| IBIS file stm32u535_545_ufbga64.ibs
[IBIS ver] 4.2
[File name] stm32u535_545_ufbga64.ibs
[File Rev] rev1.0
[Date]  11-09-2023
[Source] Data Created at STMicroelectronics
[Notes]  File originated from ELDO simulations.
[Disclaimer]  This information is for modeling purpose only and is
   not guaranteed. The information is subject to change without
   notice.
[Copyright] Copyright 2023 STMicroelectronics Inc.
|   Component stm32u535_545_ufbga64
[Component] stm32u535_545_ufbga64
[Manufacturer] STMicroelectronics
[Package]
| variable   typ   min   max
R_pkg  0  NA  NA
L_pkg  0  NA  NA
C_pkg  0  NA  NA
[Pin]   signal_name   model_name
A1  PC14-OSC32_IN   io8_100m_tamp_ft
A2  PC13  io8_100m_ft_v33
A3  PB9  io8_100m_hslv_i2c_ft
A4  PB4  io8_100m_i2c_ft
A5  PB3  io8_100m_i2c_ft
A6  PA15  io8_100m_ft
A7  PA14  io8_100m_ft
A8  PA13  io8_100m_ft
B1  PC15-OSC32_OUT  io8_100m_tamp_ft
B2  VBAT  power
B3  PB8  io8_100m_hslv_i2c_ft
B4  PH3-BOOT0  io8_100m_ft
B5  PD2  io8_100m_hslv_ft
B6  PC11  io8_100m_hslv_ft
B7  PC10  io8_100m_hslv_ft
B8  PA12  io8_usb_ft
C1  PH0-OSC_IN  io8_100m_ft
C2  VSS  gnd
C3  PB7  io8_166m_hslv_i2c_ft
C4  PB5  io8_166m_hslv_ft
C5  PC12  io8_166m_hslv_ft
C6  PA10  io8_100m_ft
C7  PA9  io8_100m_ft
C8  PA11  io8_usb_ft
D1  PH1-OSC_OUT  io8_100m_ft
D2  VDD  power
D3  PB6  io8_100m_i2c_ft
D4  VSS  gnd
D5  VSS  gnd
D6  VSS  gnd
D7  PA8  io8_166m_hslv_ft
D8  PC9  io8_100m_hslv_ft
E1  NRST  nc
E2  PC1  io8_166m_hslv_i2c_ft
E3  PC0  io8_100m_hslv_i2c_ft
E4  VDD  power
E5  VDDUSB  power
E6  VDD  power
E7  PC7  io8_100m_hslv_ft
E8  PC8  io8_100m_hslv_ft
F1  VSSA  nc
F2  PC2  io8_100m_hslv_ft
F3  PA2  io8_100m_hslv_ft
F4  PA5  io8_100m_ft
F5  PB0  io8_100m_hslv_ft
F6  PC6  io8_100m_hslv_ft
F7  PB15  io8_100m_ft
F8  PB14  io8_100m_i2c_ft
G1  PC3  io8_100m_hslv_ft
G2  PA0  io8_100m_hslv_tamp_ft
G3  PA3  io8_166m_hslv_ft
G4  PA6  io8_100m_hslv_ft
G5  PB1  io8_100m_hslv_ft
G6  PB2  io8_100m_hslv_tamp_ft
G7  PB10  io8_166m_hslv_i2c_ft
G8  PB13  io8_100m_i2c_ft
H1  VDDA  power
H2  PA1  io8_100m_hslv_tamp_ft
H3  PA4  io8_100m_hslv_ft
H4  PA7  io8_100m_hslv_i2c_ft
H5  PC4  io8_100m_hslv_ft
H6  PC5  io8_100m_tamp_ft
H7  VCAP  nc
H8  PB12  io8_166m_hslv_ft
[Package Model]   455-ufbga-5x5-64ldo-100mhz-230421
[Pin Mapping]   pulldown_ref   pullup_ref   | Comment
A1  gndio  vddiom  | Depending on IO usage
| A1  gndio  vsw  | Depending on IO usage
A2  gndio  vddiom  | Depending on IO usage
| A2  gndio  vsw  | Depending on IO usage
A3  gndio  vddiom
A4  gndio  vddiom
A5  gndio  vddiom
A6  gndio  vddiom
A7  gndio  vddiom
A8  gndio  vddiom  | Depending on IO usage
| A8  gndio  vddusb  | Depending on IO usage
B1  gndio  vddiom  | Depending on IO usage
| B1  gndio  vsw  | Depending on IO usage
B2  nc  vsw
B3  gndio  vddiom
B4  gndio  vddiom
B5  gndio  vddiom
B6  gndio  vddiom
B7  gndio  vddiom
B8  gndio  vddiom  | Depending on IO usage
| B8  gndio  vddusb  | Depending on IO usage
C1  gndio  vddiom
C2  gndio  nc
C3  gndio  vddiom
C4  gndio  vddiom
C5  gndio  vddiom
C6  gndio  vddiom  | Depending on IO usage
| C6  gndio  vddusb  | Depending on IO usage
C7  gndio  vddiom  | Depending on IO usage
| C7  gndio  vddusb  | Depending on IO usage
C8  gndio  vddiom  | Depending on IO usage
| C8  gndio  vddusb  | Depending on IO usage
D1  gndio  vddiom
D2  nc  vddiom
D3  gndio  vddiom
D4  gndio  nc
D5  gndio  nc
D6  gndio  nc
D7  gndio  vddiom
D8  gndio  vddiom
E1  nc   nc
E2  gndio  vddiom
E3  gndio  vddiom
E4  nc  vddiom
E5  nc  vddusb
E6  nc  vddiom
E7  gndio  vddiom
E8  gndio  vddiom
F1  nc  nc
F2  gndio  vddiom
F3  gndio  vddiom
F4  gndio  vddiom
F5  gndio  vddiom
F6  gndio  vddiom
F7  gndio  vddiom
F8  gndio  vddiom
G1  gndio  vddiom
G2  gndio  vddiom
G3  gndio  vddiom
G4  gndio  vddiom
G5  gndio  vddiom
G6  gndio  vddiom
G7  gndio  vddiom
G8  gndio  vddiom
H1  nc  vddiom
H2  gndio  vddiom
H3  gndio  vddiom
H4  gndio  vddiom
H5  gndio  vddiom
H6  gndio  vddiom
H7  nc  nc
H8  gndio  vddiom
[Model Selector] io8_100m_ft
io8_100m_ft_hs_1v2  "IO8_FT 100MHz high speed @ 1.2V"
io8_100m_ft_fs_1v2  "IO8_FT 100MHz fast speed @ 1.2V"
io8_100m_ft_fs_pd_1v2  "IO8_FT 100MHz fast speed @ 1.2V pulldown"
io8_100m_ft_ms_1v2  "IO8_FT 100MHz med speed @ 1.2V"
io8_100m_ft_ms_pd_1v2  "IO8_FT 100MHz med speed @ 1.2V pulldown"
io8_100m_ft_ls_1v2  "IO8_FT 100MHz low speed @ 1.2V"
io8_100m_ft_ls_pd_1v2  "IO8_FT 100MHz low speed @ 1.2V pulldown"
io8_100m_ft_hs_1v8  "IO8_FT 100MHz high speed @ 1.8V"
io8_100m_ft_hs_pd_1v8  "IO8_FT 100MHz high speed @ 1.8V pulldown"
io8_100m_ft_fs_1v8  "IO8_FT 100MHz fast speed @ 1.8V"
io8_100m_ft_fs_pd_1v8  "IO8_FT 100MHz fast speed @ 1.8V pulldown"
io8_100m_ft_ms_1v8  "IO8_FT 100MHz med speed @ 1.8V"
io8_100m_ft_ms_pd_1v8  "IO8_FT 100MHz med speed @ 1.8V pulldown"
io8_100m_ft_ls_1v8  "IO8_FT 100MHz low speed @ 1.8V"
io8_100m_ft_ls_pd_1v8  "IO8_FT 100MHz low speed @ 1.8V pulldown"
io8_100m_ft_hs_3v3  "IO8_FT 100MHz high speed @ 3.3V"
io8_100m_ft_hs_pd_3v3  "IO8_FT 100MHz high speed @ 3.3V pulldown"
io8_100m_ft_fs_3v3  "IO8_FT 100MHz fast speed @ 3.3V"
io8_100m_ft_fs_pd_3v3  "IO8_FT 100MHz fast speed @ 3.3V pulldown"
io8_100m_ft_ms_3v3  "IO8_FT 100MHz med speed @ 3.3V"
io8_100m_ft_ms_pd_3v3  "IO8_FT 100MHz med speed @ 3.3V pulldown"
io8_100m_ft_ls_3v3  "IO8_FT 100MHz low speed @ 3.3V"
io8_100m_ft_ls_pd_3v3  "IO8_FT 100MHz low speed @ 3.3V pulldown"
[Model Selector] io8_100m_hslv_ft
io8_100m_ft_hs_1v2  "IO8_FT 100MHz high speed @ 1.2V"
io8_100m_ft_hs_pu_1v2  "IO8_FT 100MHz high speed @ 1.2V pullup"
io8_100m_ft_hs_pd_1v2  "IO8_FT 100MHz high speed @ 1.2V pulldown"
io8_100m_ft_fs_1v2  "IO8_FT 100MHz fast speed @ 1.2V"
io8_100m_ft_fs_pu_1v2  "IO8_FT 100MHz fast speed @ 1.2V pullup"
io8_100m_ft_fs_pd_1v2  "IO8_FT 100MHz fast speed @ 1.2V pulldown"
io8_100m_ft_ms_1v2  "IO8_FT 100MHz med speed @ 1.2V"
io8_100m_ft_ms_pu_1v2  "IO8_FT 100MHz med speed @ 1.2V pullup"
io8_100m_ft_ms_pd_1v2  "IO8_FT 100MHz med speed @ 1.2V pulldown"
io8_100m_ft_ls_1v2  "IO8_FT 100MHz low speed @ 1.2V"
io8_100m_ft_ls_pu_1v2  "IO8_FT 100MHz low speed @ 1.2V pullup"
io8_100m_ft_ls_pd_1v2  "IO8_FT 100MHz low speed @ 1.2V pulldown"
io8_100m_ft_hs_1v8  "IO8_FT 100MHz high speed @ 1.8V"
io8_100m_ft_hs_pu_1v8  "IO8_FT 100MHz high speed @ 1.8V pullup"
io8_100m_ft_hs_pd_1v8  "IO8_FT 100MHz high speed @ 1.8V pulldown"
io8_100m_ft_fs_1v8  "IO8_FT 100MHz fast speed @ 1.8V"
io8_100m_ft_fs_pu_1v8  "IO8_FT 100MHz fast speed @ 1.8V pullup"
io8_100m_ft_fs_pd_1v8  "IO8_FT 100MHz fast speed @ 1.8V pulldown"
io8_100m_ft_ms_1v8  "IO8_FT 100MHz med speed @ 1.8V"
io8_100m_ft_ms_pu_1v8  "IO8_FT 100MHz med speed @ 1.8V pullup"
io8_100m_ft_ms_pd_1v8  "IO8_FT 100MHz med speed @ 1.8V pulldown"
io8_100m_ft_ls_1v8  "IO8_FT 100MHz low speed @ 1.8V"
io8_100m_ft_ls_pu_1v8  "IO8_FT 100MHz low speed @ 1.8V pullup"
io8_100m_ft_ls_pd_1v8  "IO8_FT 100MHz low speed @ 1.8V pulldown"
io8_100m_ft_hs_3v3  "IO8_FT 100MHz high speed @ 3.3V"
io8_100m_ft_hs_pu_3v3  "IO8_FT 100MHz high speed @ 3.3V pullup"
io8_100m_ft_hs_pd_3v3  "IO8_FT 100MHz high speed @ 3.3V pulldown"
io8_100m_ft_fs_3v3  "IO8_FT 100MHz fast speed @ 3.3V"
io8_100m_ft_fs_pu_3v3  "IO8_FT 100MHz fast speed @ 3.3V pullup"
io8_100m_ft_fs_pd_3v3  "IO8_FT 100MHz fast speed @ 3.3V pulldown"
io8_100m_ft_ms_3v3  "IO8_FT 100MHz med speed @ 3.3V"
io8_100m_ft_ms_pu_3v3  "IO8_FT 100MHz med speed @ 3.3V pullup"
io8_100m_ft_ms_pd_3v3  "IO8_FT 100MHz med speed @ 3.3V pulldown"
io8_100m_ft_ls_3v3  "IO8_FT 100MHz low speed @ 3.3V"
io8_100m_ft_ls_pu_3v3  "IO8_FT 100MHz low speed @ 3.3V pullup"
io8_100m_ft_ls_pd_3v3  "IO8_FT 100MHz low speed @ 3.3V pulldown"
io8_100m_hslv_ft_hs_1v2  "IO8_FT 100MHz HSLV high speed @ 1.2V"
io8_100m_hslv_ft_hs_pu_1v2  "IO8_FT 100MHz HSLV high speed @ 1.2V pullup"
io8_100m_hslv_ft_hs_pd_1v2  "IO8_FT 100MHz HSLV high speed @ 1.2V pulldown"
io8_100m_hslv_ft_fs_1v2  "IO8_FT 100MHz HSLV fast speed @ 1.2V"
io8_100m_hslv_ft_fs_pu_1v2  "IO8_FT 100MHz HSLV fast speed @ 1.2V pullup"
io8_100m_hslv_ft_fs_pd_1v2  "IO8_FT 100MHz HSLV fast speed @ 1.2V pulldown"
io8_100m_hslv_ft_ms_1v2  "IO8_FT 100MHz HSLV med speed @ 1.2V"
io8_100m_hslv_ft_ms_pu_1v2  "IO8_FT 100MHz HSLV med speed @ 1.2V pullup"
io8_100m_hslv_ft_ms_pd_1v2  "IO8_FT 100MHz HSLV med speed @ 1.2V pulldown"
io8_100m_hslv_ft_ls_1v2  "IO8_FT 100MHz HSLV low speed @ 1.2V"
io8_100m_hslv_ft_ls_pu_1v2  "IO8_FT 100MHz HSLV low speed @ 1.2V pullup"
io8_100m_hslv_ft_ls_pd_1v2  "IO8_FT 100MHz HSLV low speed @ 1.2V pulldown"
io8_100m_hslv_ft_hs_1v8  "IO8_FT 100MHz HSLV high speed @ 1.8V"
io8_100m_hslv_ft_hs_pu_1v8  "IO8_FT 100MHz HSLV high speed @ 1.8V pullup"
io8_100m_hslv_ft_hs_pd_1v8  "IO8_FT 100MHz HSLV high speed @ 1.8V pulldown"
io8_100m_hslv_ft_fs_1v8  "IO8_FT 100MHz HSLV fast speed @ 1.8V"
io8_100m_hslv_ft_fs_pu_1v8  "IO8_FT 100MHz HSLV fast speed @ 1.8V pullup"
io8_100m_hslv_ft_fs_pd_1v8  "IO8_FT 100MHz HSLV fast speed @ 1.8V pulldown"
io8_100m_hslv_ft_ms_1v8  "IO8_FT 100MHz HSLV med speed @ 1.8V"
io8_100m_hslv_ft_ms_pu_1v8  "IO8_FT 100MHz HSLV med speed @ 1.8V pullup"
io8_100m_hslv_ft_ms_pd_1v8  "IO8_FT 100MHz HSLV med speed @ 1.8V pulldown"
io8_100m_hslv_ft_ls_1v8  "IO8_FT 100MHz HSLV low speed @ 1.8V"
io8_100m_hslv_ft_ls_pu_1v8  "IO8_FT 100MHz HSLV low speed @ 1.8V pullup"
io8_100m_hslv_ft_ls_pd_1v8  "IO8_FT 100MHz HSLV low speed @ 1.8V pulldown"
io8_100m_hslv_ft_hs_2v5  "IO8_FT 100MHz HSLV high speed @ 2.5V"
io8_100m_hslv_ft_hs_pu_2v5  "IO8_FT 100MHz HSLV high speed @ 2.5V pullup"
io8_100m_hslv_ft_hs_pd_2v5  "IO8_FT 100MHz HSLV high speed @ 2.5V pulldown"
io8_100m_hslv_ft_fs_2v5  "IO8_FT 100MHz HSLV fast speed @ 2.5V"
io8_100m_hslv_ft_fs_pu_2v5  "IO8_FT 100MHz HSLV fast speed @ 2.5V pullup"
io8_100m_hslv_ft_fs_pd_2v5  "IO8_FT 100MHz HSLV fast speed @ 2.5V pulldown"
io8_100m_hslv_ft_ms_2v5  "IO8_FT 100MHz HSLV med speed @ 2.5V"
io8_100m_hslv_ft_ms_pu_2v5  "IO8_FT 100MHz HSLV med speed @ 2.5V pullup"
io8_100m_hslv_ft_ms_pd_2v5  "IO8_FT 100MHz HSLV med speed @ 2.5V pulldown"
io8_100m_hslv_ft_ls_2v5  "IO8_FT 100MHz HSLV low speed @ 2.5V"
io8_100m_hslv_ft_ls_pu_2v5  "IO8_FT 100MHz HSLV low speed @ 2.5V pullup"
io8_100m_hslv_ft_ls_pd_2v5  "IO8_FT 100MHz HSLV low speed @ 2.5V pulldown"
[Model Selector] io8_100m_hslv_i2c_ft
io8_100m_ft_hs_1v2  "IO8_FT 100MHz high speed @ 1.2V"
io8_100m_ft_hs_pu_1v2  "IO8_FT 100MHz high speed @ 1.2V pullup"
io8_100m_ft_hs_pd_1v2  "IO8_FT 100MHz high speed @ 1.2V pulldown"
io8_100m_ft_fs_1v2  "IO8_FT 100MHz fast speed @ 1.2V"
io8_100m_ft_fs_pu_1v2  "IO8_FT 100MHz fast speed @ 1.2V pullup"
io8_100m_ft_fs_pd_1v2  "IO8_FT 100MHz fast speed @ 1.2V pulldown"
io8_100m_ft_ms_1v2  "IO8_FT 100MHz med speed @ 1.2V"
io8_100m_ft_ms_pu_1v2  "IO8_FT 100MHz med speed @ 1.2V pullup"
io8_100m_ft_ms_pd_1v2  "IO8_FT 100MHz med speed @ 1.2V pulldown"
io8_100m_ft_ls_1v2  "IO8_FT 100MHz low speed @ 1.2V"
io8_100m_ft_ls_pu_1v2  "IO8_FT 100MHz low speed @ 1.2V pullup"
io8_100m_ft_ls_pd_1v2  "IO8_FT 100MHz low speed @ 1.2V pulldown"
io8_100m_ft_hs_1v8  "IO8_FT 100MHz high speed @ 1.8V"
io8_100m_ft_hs_pu_1v8  "IO8_FT 100MHz high speed @ 1.8V pullup"
io8_100m_ft_hs_pd_1v8  "IO8_FT 100MHz high speed @ 1.8V pulldown"
io8_100m_ft_fs_1v8  "IO8_FT 100MHz fast speed @ 1.8V"
io8_100m_ft_fs_pu_1v8  "IO8_FT 100MHz fast speed @ 1.8V pullup"
io8_100m_ft_fs_pd_1v8  "IO8_FT 100MHz fast speed @ 1.8V pulldown"
io8_100m_ft_ms_1v8  "IO8_FT 100MHz med speed @ 1.8V"
io8_100m_ft_ms_pu_1v8  "IO8_FT 100MHz med speed @ 1.8V pullup"
io8_100m_ft_ms_pd_1v8  "IO8_FT 100MHz med speed @ 1.8V pulldown"
io8_100m_ft_ls_1v8  "IO8_FT 100MHz low speed @ 1.8V"
io8_100m_ft_ls_pu_1v8  "IO8_FT 100MHz low speed @ 1.8V pullup"
io8_100m_ft_ls_pd_1v8  "IO8_FT 100MHz low speed @ 1.8V pulldown"
io8_100m_ft_hs_3v3  "IO8_FT 100MHz high speed @ 3.3V"
io8_100m_ft_hs_pu_3v3  "IO8_FT 100MHz high speed @ 3.3V pullup"
io8_100m_ft_hs_pd_3v3  "IO8_FT 100MHz high speed @ 3.3V pulldown"
io8_100m_ft_fs_3v3  "IO8_FT 100MHz fast speed @ 3.3V"
io8_100m_ft_fs_pu_3v3  "IO8_FT 100MHz fast speed @ 3.3V pullup"
io8_100m_ft_fs_pd_3v3  "IO8_FT 100MHz fast speed @ 3.3V pulldown"
io8_100m_ft_ms_3v3  "IO8_FT 100MHz med speed @ 3.3V"
io8_100m_ft_ms_pu_3v3  "IO8_FT 100MHz med speed @ 3.3V pullup"
io8_100m_ft_ms_pd_3v3  "IO8_FT 100MHz med speed @ 3.3V pulldown"
io8_100m_ft_ls_3v3  "IO8_FT 100MHz low speed @ 3.3V"
io8_100m_ft_ls_pu_3v3  "IO8_FT 100MHz low speed @ 3.3V pullup"
io8_100m_ft_ls_pd_3v3  "IO8_FT 100MHz low speed @ 3.3V pulldown"
io8_100m_hslv_ft_hs_1v2  "IO8_FT 100MHz HSLV high speed @ 1.2V"
io8_100m_hslv_ft_hs_pu_1v2  "IO8_FT 100MHz HSLV high speed @ 1.2V pullup"
io8_100m_hslv_ft_hs_pd_1v2  "IO8_FT 100MHz HSLV high speed @ 1.2V pulldown"
io8_100m_hslv_ft_fs_1v2  "IO8_FT 100MHz HSLV fast speed @ 1.2V"
io8_100m_hslv_ft_fs_pu_1v2  "IO8_FT 100MHz HSLV fast speed @ 1.2V pullup"
io8_100m_hslv_ft_fs_pd_1v2  "IO8_FT 100MHz HSLV fast speed @ 1.2V pulldown"
io8_100m_hslv_ft_ms_1v2  "IO8_FT 100MHz HSLV med speed @ 1.2V"
io8_100m_hslv_ft_ms_pu_1v2  "IO8_FT 100MHz HSLV med speed @ 1.2V pullup"
io8_100m_hslv_ft_ms_pd_1v2  "IO8_FT 100MHz HSLV med speed @ 1.2V pulldown"
io8_100m_hslv_ft_ls_1v2  "IO8_FT 100MHz HSLV low speed @ 1.2V"
io8_100m_hslv_ft_ls_pu_1v2  "IO8_FT 100MHz HSLV low speed @ 1.2V pullup"
io8_100m_hslv_ft_ls_pd_1v2  "IO8_FT 100MHz HSLV low speed @ 1.2V pulldown"
io8_100m_hslv_ft_hs_1v8  "IO8_FT 100MHz HSLV high speed @ 1.8V"
io8_100m_hslv_ft_hs_pu_1v8  "IO8_FT 100MHz HSLV high speed @ 1.8V pullup"
io8_100m_hslv_ft_hs_pd_1v8  "IO8_FT 100MHz HSLV high speed @ 1.8V pulldown"
io8_100m_hslv_ft_fs_1v8  "IO8_FT 100MHz HSLV fast speed @ 1.8V"
io8_100m_hslv_ft_fs_pu_1v8  "IO8_FT 100MHz HSLV fast speed @ 1.8V pullup"
io8_100m_hslv_ft_fs_pd_1v8  "IO8_FT 100MHz HSLV fast speed @ 1.8V pulldown"
io8_100m_hslv_ft_ms_1v8  "IO8_FT 100MHz HSLV med speed @ 1.8V"
io8_100m_hslv_ft_ms_pu_1v8  "IO8_FT 100MHz HSLV med speed @ 1.8V pullup"
io8_100m_hslv_ft_ms_pd_1v8  "IO8_FT 100MHz HSLV med speed @ 1.8V pulldown"
io8_100m_hslv_ft_ls_1v8  "IO8_FT 100MHz HSLV low speed @ 1.8V"
io8_100m_hslv_ft_ls_pu_1v8  "IO8_FT 100MHz HSLV low speed @ 1.8V pullup"
io8_100m_hslv_ft_ls_pd_1v8  "IO8_FT 100MHz HSLV low speed @ 1.8V pulldown"
io8_100m_hslv_ft_hs_2v5  "IO8_FT 100MHz HSLV high speed @ 2.5V"
io8_100m_hslv_ft_hs_pu_2v5  "IO8_FT 100MHz HSLV high speed @ 2.5V pullup"
io8_100m_hslv_ft_hs_pd_2v5  "IO8_FT 100MHz HSLV high speed @ 2.5V pulldown"
io8_100m_hslv_ft_fs_2v5  "IO8_FT 100MHz HSLV fast speed @ 2.5V"
io8_100m_hslv_ft_fs_pu_2v5  "IO8_FT 100MHz HSLV fast speed @ 2.5V pullup"
io8_100m_hslv_ft_fs_pd_2v5  "IO8_FT 100MHz HSLV fast speed @ 2.5V pulldown"
io8_100m_hslv_ft_ms_2v5  "IO8_FT 100MHz HSLV med speed @ 2.5V"
io8_100m_hslv_ft_ms_pu_2v5  "IO8_FT 100MHz HSLV med speed @ 2.5V pullup"
io8_100m_hslv_ft_ms_pd_2v5  "IO8_FT 100MHz HSLV med speed @ 2.5V pulldown"
io8_100m_hslv_ft_ls_2v5  "IO8_FT 100MHz HSLV low speed @ 2.5V"
io8_100m_hslv_ft_ls_pu_2v5  "IO8_FT 100MHz HSLV low speed @ 2.5V pullup"
io8_100m_hslv_ft_ls_pd_2v5  "IO8_FT 100MHz HSLV low speed @ 2.5V pulldown"
[Model Selector] io8_100m_hslv_tamp_ft
io8_100m_ft_hs_1v2  "IO8_FT 100MHz high speed @ 1.2V"
io8_100m_ft_hs_pu_1v2  "IO8_FT 100MHz high speed @ 1.2V pullup"
io8_100m_ft_hs_pd_1v2  "IO8_FT 100MHz high speed @ 1.2V pulldown"
io8_100m_ft_fs_1v2  "IO8_FT 100MHz fast speed @ 1.2V"
io8_100m_ft_fs_pu_1v2  "IO8_FT 100MHz fast speed @ 1.2V pullup"
io8_100m_ft_fs_pd_1v2  "IO8_FT 100MHz fast speed @ 1.2V pulldown"
io8_100m_ft_ms_1v2  "IO8_FT 100MHz med speed @ 1.2V"
io8_100m_ft_ms_pu_1v2  "IO8_FT 100MHz med speed @ 1.2V pullup"
io8_100m_ft_ms_pd_1v2  "IO8_FT 100MHz med speed @ 1.2V pulldown"
io8_100m_ft_ls_1v2  "IO8_FT 100MHz low speed @ 1.2V"
io8_100m_ft_ls_pu_1v2  "IO8_FT 100MHz low speed @ 1.2V pullup"
io8_100m_ft_ls_pd_1v2  "IO8_FT 100MHz low speed @ 1.2V pulldown"
io8_100m_ft_hs_1v8  "IO8_FT 100MHz high speed @ 1.8V"
io8_100m_ft_hs_pu_1v8  "IO8_FT 100MHz high speed @ 1.8V pullup"
io8_100m_ft_hs_pd_1v8  "IO8_FT 100MHz high speed @ 1.8V pulldown"
io8_100m_ft_fs_1v8  "IO8_FT 100MHz fast speed @ 1.8V"
io8_100m_ft_fs_pu_1v8  "IO8_FT 100MHz fast speed @ 1.8V pullup"
io8_100m_ft_fs_pd_1v8  "IO8_FT 100MHz fast speed @ 1.8V pulldown"
io8_100m_ft_ms_1v8  "IO8_FT 100MHz med speed @ 1.8V"
io8_100m_ft_ms_pu_1v8  "IO8_FT 100MHz med speed @ 1.8V pullup"
io8_100m_ft_ms_pd_1v8  "IO8_FT 100MHz med speed @ 1.8V pulldown"
io8_100m_ft_ls_1v8  "IO8_FT 100MHz low speed @ 1.8V"
io8_100m_ft_ls_pu_1v8  "IO8_FT 100MHz low speed @ 1.8V pullup"
io8_100m_ft_ls_pd_1v8  "IO8_FT 100MHz low speed @ 1.8V pulldown"
io8_100m_ft_hs_3v3  "IO8_FT 100MHz high speed @ 3.3V"
io8_100m_ft_hs_pu_3v3  "IO8_FT 100MHz high speed @ 3.3V pullup"
io8_100m_ft_hs_pd_3v3  "IO8_FT 100MHz high speed @ 3.3V pulldown"
io8_100m_ft_fs_3v3  "IO8_FT 100MHz fast speed @ 3.3V"
io8_100m_ft_fs_pu_3v3  "IO8_FT 100MHz fast speed @ 3.3V pullup"
io8_100m_ft_fs_pd_3v3  "IO8_FT 100MHz fast speed @ 3.3V pulldown"
io8_100m_ft_ms_3v3  "IO8_FT 100MHz med speed @ 3.3V"
io8_100m_ft_ms_pu_3v3  "IO8_FT 100MHz med speed @ 3.3V pullup"
io8_100m_ft_ms_pd_3v3  "IO8_FT 100MHz med speed @ 3.3V pulldown"
io8_100m_ft_ls_3v3  "IO8_FT 100MHz low speed @ 3.3V"
io8_100m_ft_ls_pu_3v3  "IO8_FT 100MHz low speed @ 3.3V pullup"
io8_100m_ft_ls_pd_3v3  "IO8_FT 100MHz low speed @ 3.3V pulldown"
io8_100m_hslv_ft_hs_1v2  "IO8_FT 100MHz HSLV high speed @ 1.2V"
io8_100m_hslv_ft_hs_pu_1v2  "IO8_FT 100MHz HSLV high speed @ 1.2V pullup"
io8_100m_hslv_ft_hs_pd_1v2  "IO8_FT 100MHz HSLV high speed @ 1.2V pulldown"
io8_100m_hslv_ft_fs_1v2  "IO8_FT 100MHz HSLV fast speed @ 1.2V"
io8_100m_hslv_ft_fs_pu_1v2  "IO8_FT 100MHz HSLV fast speed @ 1.2V pullup"
io8_100m_hslv_ft_fs_pd_1v2  "IO8_FT 100MHz HSLV fast speed @ 1.2V pulldown"
io8_100m_hslv_ft_ms_1v2  "IO8_FT 100MHz HSLV med speed @ 1.2V"
io8_100m_hslv_ft_ms_pu_1v2  "IO8_FT 100MHz HSLV med speed @ 1.2V pullup"
io8_100m_hslv_ft_ms_pd_1v2  "IO8_FT 100MHz HSLV med speed @ 1.2V pulldown"
io8_100m_hslv_ft_ls_1v2  "IO8_FT 100MHz HSLV low speed @ 1.2V"
io8_100m_hslv_ft_ls_pu_1v2  "IO8_FT 100MHz HSLV low speed @ 1.2V pullup"
io8_100m_hslv_ft_ls_pd_1v2  "IO8_FT 100MHz HSLV low speed @ 1.2V pulldown"
io8_100m_hslv_ft_hs_1v8  "IO8_FT 100MHz HSLV high speed @ 1.8V"
io8_100m_hslv_ft_hs_pu_1v8  "IO8_FT 100MHz HSLV high speed @ 1.8V pullup"
io8_100m_hslv_ft_hs_pd_1v8  "IO8_FT 100MHz HSLV high speed @ 1.8V pulldown"
io8_100m_hslv_ft_fs_1v8  "IO8_FT 100MHz HSLV fast speed @ 1.8V"
io8_100m_hslv_ft_fs_pu_1v8  "IO8_FT 100MHz HSLV fast speed @ 1.8V pullup"
io8_100m_hslv_ft_fs_pd_1v8  "IO8_FT 100MHz HSLV fast speed @ 1.8V pulldown"
io8_100m_hslv_ft_ms_1v8  "IO8_FT 100MHz HSLV med speed @ 1.8V"
io8_100m_hslv_ft_ms_pu_1v8  "IO8_FT 100MHz HSLV med speed @ 1.8V pullup"
io8_100m_hslv_ft_ms_pd_1v8  "IO8_FT 100MHz HSLV med speed @ 1.8V pulldown"
io8_100m_hslv_ft_ls_1v8  "IO8_FT 100MHz HSLV low speed @ 1.8V"
io8_100m_hslv_ft_ls_pu_1v8  "IO8_FT 100MHz HSLV low speed @ 1.8V pullup"
io8_100m_hslv_ft_ls_pd_1v8  "IO8_FT 100MHz HSLV low speed @ 1.8V pulldown"
io8_100m_hslv_ft_hs_2v5  "IO8_FT 100MHz HSLV high speed @ 2.5V"
io8_100m_hslv_ft_hs_pu_2v5  "IO8_FT 100MHz HSLV high speed @ 2.5V pullup"
io8_100m_hslv_ft_hs_pd_2v5  "IO8_FT 100MHz HSLV high speed @ 2.5V pulldown"
io8_100m_hslv_ft_fs_2v5  "IO8_FT 100MHz HSLV fast speed @ 2.5V"
io8_100m_hslv_ft_fs_pu_2v5  "IO8_FT 100MHz HSLV fast speed @ 2.5V pullup"
io8_100m_hslv_ft_fs_pd_2v5  "IO8_FT 100MHz HSLV fast speed @ 2.5V pulldown"
io8_100m_hslv_ft_ms_2v5  "IO8_FT 100MHz HSLV med speed @ 2.5V"
io8_100m_hslv_ft_ms_pu_2v5  "IO8_FT 100MHz HSLV med speed @ 2.5V pullup"
io8_100m_hslv_ft_ms_pd_2v5  "IO8_FT 100MHz HSLV med speed @ 2.5V pulldown"
io8_100m_hslv_ft_ls_2v5  "IO8_FT 100MHz HSLV low speed @ 2.5V"
io8_100m_hslv_ft_ls_pu_2v5  "IO8_FT 100MHz HSLV low speed @ 2.5V pullup"
io8_100m_hslv_ft_ls_pd_2v5  "IO8_FT 100MHz HSLV low speed @ 2.5V pulldown"
io8_ft_v33_hs_1v2  "IO8_FT_V33 high speed @ 1.2V"
io8_ft_v33_hs_pu_1v2  "IO8_FT_V33 high speed @ 1.2V pullup"
io8_ft_v33_hs_pd_1v2  "IO8_FT_V33 high speed @ 1.2V pulldown"
io8_ft_v33_fs_1v2  "IO8_FT_V33 fast speed @ 1.2V"
io8_ft_v33_fs_pu_1v2  "IO8_FT_V33 fast speed @ 1.2V pullup"
io8_ft_v33_fs_pd_1v2  "IO8_FT_V33 fast speed @ 1.2V pulldown"
io8_ft_v33_ms_1v2  "IO8_FT_V33 med speed @ 1.2V"
io8_ft_v33_ms_pu_1v2  "IO8_FT_V33 med speed @ 1.2V pullup"
io8_ft_v33_ms_pd_1v2  "IO8_FT_V33 med speed @ 1.2V pulldown"
io8_ft_v33_ls_1v2  "IO8_FT_V33 low speed @ 1.2V"
io8_ft_v33_ls_pu_1v2  "IO8_FT_V33 low speed @ 1.2V pullup"
io8_ft_v33_ls_pd_1v2  "IO8_FT_V33 low speed @ 1.2V pulldown"
io8_ft_v33_hs_1v8  "IO8_FT_V33 high speed @ 1.8V"
io8_ft_v33_hs_pu_1v8  "IO8_FT_V33 high speed @ 1.8V pullup"
io8_ft_v33_hs_pd_1v8  "IO8_FT_V33 high speed @ 1.8V pulldown"
io8_ft_v33_fs_1v8  "IO8_FT_V33 fast speed @ 1.8V"
io8_ft_v33_fs_pu_1v8  "IO8_FT_V33 fast speed @ 1.8V pullup"
io8_ft_v33_fs_pd_1v8  "IO8_FT_V33 fast speed @ 1.8V pulldown"
io8_ft_v33_ms_1v8  "IO8_FT_V33 med speed @ 1.8V"
io8_ft_v33_ms_pu_1v8  "IO8_FT_V33 med speed @ 1.8V pullup"
io8_ft_v33_ms_pd_1v8  "IO8_FT_V33 med speed @ 1.8V pulldown"
io8_ft_v33_ls_1v8  "IO8_FT_V33 low speed @ 1.8V"
io8_ft_v33_ls_pu_1v8  "IO8_FT_V33 low speed @ 1.8V pullup"
io8_ft_v33_ls_pd_1v8  "IO8_FT_V33 low speed @ 1.8V pulldown"
io8_ft_v33_hs_3v3  "IO8_FT_V33 high speed @ 3.3V"
io8_ft_v33_hs_pu_3v3  "IO8_FT_V33 high speed @ 3.3V pullup"
io8_ft_v33_hs_pd_3v3  "IO8_FT_V33 high speed @ 3.3V pulldown"
io8_ft_v33_fs_3v3  "IO8_FT_V33 fast speed @ 3.3V"
io8_ft_v33_fs_pu_3v3  "IO8_FT_V33 fast speed @ 3.3V pullup"
io8_ft_v33_fs_pd_3v3  "IO8_FT_V33 fast speed @ 3.3V pulldown"
io8_ft_v33_ms_3v3  "IO8_FT_V33 med speed @ 3.3V"
io8_ft_v33_ms_pu_3v3  "IO8_FT_V33 med speed @ 3.3V pullup"
io8_ft_v33_ms_pd_3v3  "IO8_FT_V33 med speed @ 3.3V pulldown"
io8_ft_v33_ls_3v3  "IO8_FT_V33 low speed @ 3.3V"
io8_ft_v33_ls_pu_3v3  "IO8_FT_V33 low speed @ 3.3V pullup"
io8_ft_v33_ls_pd_3v3  "IO8_FT_V33 low speed @ 3.3V pulldown"
[Model Selector] io8_100m_i2c_ft
io8_100m_ft_hs_1v2  "IO8_FT 100MHz high speed @ 1.2V"
io8_100m_ft_hs_pu_1v2  "IO8_FT 100MHz high speed @ 1.2V pullup"
io8_100m_ft_hs_pd_1v2  "IO8_FT 100MHz high speed @ 1.2V pulldown"
io8_100m_ft_fs_1v2  "IO8_FT 100MHz fast speed @ 1.2V"
io8_100m_ft_fs_pu_1v2  "IO8_FT 100MHz fast speed @ 1.2V pullup"
io8_100m_ft_fs_pd_1v2  "IO8_FT 100MHz fast speed @ 1.2V pulldown"
io8_100m_ft_ms_1v2  "IO8_FT 100MHz med speed @ 1.2V"
io8_100m_ft_ms_pu_1v2  "IO8_FT 100MHz med speed @ 1.2V pullup"
io8_100m_ft_ms_pd_1v2  "IO8_FT 100MHz med speed @ 1.2V pulldown"
io8_100m_ft_ls_1v2  "IO8_FT 100MHz low speed @ 1.2V"
io8_100m_ft_ls_pu_1v2  "IO8_FT 100MHz low speed @ 1.2V pullup"
io8_100m_ft_ls_pd_1v2  "IO8_FT 100MHz low speed @ 1.2V pulldown"
io8_100m_ft_hs_1v8  "IO8_FT 100MHz high speed @ 1.8V"
io8_100m_ft_hs_pu_1v8  "IO8_FT 100MHz high speed @ 1.8V pullup"
io8_100m_ft_hs_pd_1v8  "IO8_FT 100MHz high speed @ 1.8V pulldown"
io8_100m_ft_fs_1v8  "IO8_FT 100MHz fast speed @ 1.8V"
io8_100m_ft_fs_pu_1v8  "IO8_FT 100MHz fast speed @ 1.8V pullup"
io8_100m_ft_fs_pd_1v8  "IO8_FT 100MHz fast speed @ 1.8V pulldown"
io8_100m_ft_ms_1v8  "IO8_FT 100MHz med speed @ 1.8V"
io8_100m_ft_ms_pu_1v8  "IO8_FT 100MHz med speed @ 1.8V pullup"
io8_100m_ft_ms_pd_1v8  "IO8_FT 100MHz med speed @ 1.8V pulldown"
io8_100m_ft_ls_1v8  "IO8_FT 100MHz low speed @ 1.8V"
io8_100m_ft_ls_pu_1v8  "IO8_FT 100MHz low speed @ 1.8V pullup"
io8_100m_ft_ls_pd_1v8  "IO8_FT 100MHz low speed @ 1.8V pulldown"
io8_100m_ft_hs_3v3  "IO8_FT 100MHz high speed @ 3.3V"
io8_100m_ft_hs_pu_3v3  "IO8_FT 100MHz high speed @ 3.3V pullup"
io8_100m_ft_hs_pd_3v3  "IO8_FT 100MHz high speed @ 3.3V pulldown"
io8_100m_ft_fs_3v3  "IO8_FT 100MHz fast speed @ 3.3V"
io8_100m_ft_fs_pu_3v3  "IO8_FT 100MHz fast speed @ 3.3V pullup"
io8_100m_ft_fs_pd_3v3  "IO8_FT 100MHz fast speed @ 3.3V pulldown"
io8_100m_ft_ms_3v3  "IO8_FT 100MHz med speed @ 3.3V"
io8_100m_ft_ms_pu_3v3  "IO8_FT 100MHz med speed @ 3.3V pullup"
io8_100m_ft_ms_pd_3v3  "IO8_FT 100MHz med speed @ 3.3V pulldown"
io8_100m_ft_ls_3v3  "IO8_FT 100MHz low speed @ 3.3V"
io8_100m_ft_ls_pu_3v3  "IO8_FT 100MHz low speed @ 3.3V pullup"
io8_100m_ft_ls_pd_3v3  "IO8_FT 100MHz low speed @ 3.3V pulldown"
io8_100m_i2c_ft_1v2  "IO8_FT 100MHz I2C @ 1.2V"
io8_100m_i2c_ft_pu_1v2  "IO8_FT 100MHz I2C @ 1.2V pullup"
io8_100m_i2c_ft_pd_1v2  "IO8_FT 100MHz I2C @ 1.2V pulldown"
io8_100m_i2c_ft_1v8  "IO8_FT 100MHz I2C @ 1.8V"
io8_100m_i2c_ft_pu_1v8  "IO8_FT 100MHz I2C @ 1.8V pullup"
io8_100m_i2c_ft_pd_1v8  "IO8_FT 100MHz I2C @ 1,8V pulldown"
io8_100m_i2c_ft_3v3  "IO8_FT 100MHz I2C @ 3.3V"
io8_100m_i2c_ft_pu_3v3  "IO8_FT 100MHz I2C HSLV @ 3.3V pullup"
io8_100m_i2c_ft_pd_3v3  "IO8_FT 100MHz I2C @ 3.3V pulldown"
[Model Selector] io8_100m_tamp_ft
io8_100m_ft_hs_1v2  "IO8_FT 100MHz high speed @ 1.2V"
io8_100m_ft_hs_pu_1v2  "IO8_FT 100MHz high speed @ 1.2V pullup"
io8_100m_ft_hs_pd_1v2  "IO8_FT 100MHz high speed @ 1.2V pulldown"
io8_100m_ft_fs_1v2  "IO8_FT 100MHz fast speed @ 1.2V"
io8_100m_ft_fs_pu_1v2  "IO8_FT 100MHz fast speed @ 1.2V pullup"
io8_100m_ft_fs_pd_1v2  "IO8_FT 100MHz fast speed @ 1.2V pulldown"
io8_100m_ft_ms_1v2  "IO8_FT 100MHz med speed @ 1.2V"
io8_100m_ft_ms_pu_1v2  "IO8_FT 100MHz med speed @ 1.2V pullup"
io8_100m_ft_ms_pd_1v2  "IO8_FT 100MHz med speed @ 1.2V pulldown"
io8_100m_ft_ls_1v2  "IO8_FT 100MHz low speed @ 1.2V"
io8_100m_ft_ls_pu_1v2  "IO8_FT 100MHz low speed @ 1.2V pullup"
io8_100m_ft_ls_pd_1v2  "IO8_FT 100MHz low speed @ 1.2V pulldown"
io8_100m_ft_hs_1v8  "IO8_FT 100MHz high speed @ 1.8V"
io8_100m_ft_hs_pu_1v8  "IO8_FT 100MHz high speed @ 1.8V pullup"
io8_100m_ft_hs_pd_1v8  "IO8_FT 100MHz high speed @ 1.8V pulldown"
io8_100m_ft_fs_1v8  "IO8_FT 100MHz fast speed @ 1.8V"
io8_100m_ft_fs_pu_1v8  "IO8_FT 100MHz fast speed @ 1.8V pullup"
io8_100m_ft_fs_pd_1v8  "IO8_FT 100MHz fast speed @ 1.8V pulldown"
io8_100m_ft_ms_1v8  "IO8_FT 100MHz med speed @ 1.8V"
io8_100m_ft_ms_pu_1v8  "IO8_FT 100MHz med speed @ 1.8V pullup"
io8_100m_ft_ms_pd_1v8  "IO8_FT 100MHz med speed @ 1.8V pulldown"
io8_100m_ft_ls_1v8  "IO8_FT 100MHz low speed @ 1.8V"
io8_100m_ft_ls_pu_1v8  "IO8_FT 100MHz low speed @ 1.8V pullup"
io8_100m_ft_ls_pd_1v8  "IO8_FT 100MHz low speed @ 1.8V pulldown"
io8_100m_ft_hs_3v3  "IO8_FT 100MHz high speed @ 3.3V"
io8_100m_ft_hs_pu_3v3  "IO8_FT 100MHz high speed @ 3.3V pullup"
io8_100m_ft_hs_pd_3v3  "IO8_FT 100MHz high speed @ 3.3V pulldown"
io8_100m_ft_fs_3v3  "IO8_FT 100MHz fast speed @ 3.3V"
io8_100m_ft_fs_pu_3v3  "IO8_FT 100MHz fast speed @ 3.3V pullup"
io8_100m_ft_fs_pd_3v3  "IO8_FT 100MHz fast speed @ 3.3V pulldown"
io8_100m_ft_ms_3v3  "IO8_FT 100MHz med speed @ 3.3V"
io8_100m_ft_ms_pu_3v3  "IO8_FT 100MHz med speed @ 3.3V pullup"
io8_100m_ft_ms_pd_3v3  "IO8_FT 100MHz med speed @ 3.3V pulldown"
io8_100m_ft_ls_3v3  "IO8_FT 100MHz low speed @ 3.3V"
io8_100m_ft_ls_pu_3v3  "IO8_FT 100MHz low speed @ 3.3V pullup"
io8_100m_ft_ls_pd_3v3  "IO8_FT 100MHz low speed @ 3.3V pulldown"
io8_ft_v33_hs_1v2  "IO8_FT_V33 high speed @ 1.2V"
io8_ft_v33_hs_pu_1v2  "IO8_FT_V33 high speed @ 1.2V pullup"
io8_ft_v33_hs_pd_1v2  "IO8_FT_V33 high speed @ 1.2V pulldown"
io8_ft_v33_fs_1v2  "IO8_FT_V33 fast speed @ 1.2V"
io8_ft_v33_fs_pu_1v2  "IO8_FT_V33 fast speed @ 1.2V pullup"
io8_ft_v33_fs_pd_1v2  "IO8_FT_V33 fast speed @ 1.2V pulldown"
io8_ft_v33_ms_1v2  "IO8_FT_V33 med speed @ 1.2V"
io8_ft_v33_ms_pu_1v2  "IO8_FT_V33 med speed @ 1.2V pullup"
io8_ft_v33_ms_pd_1v2  "IO8_FT_V33 med speed @ 1.2V pulldown"
io8_ft_v33_ls_1v2  "IO8_FT_V33 low speed @ 1.2V"
io8_ft_v33_ls_pu_1v2  "IO8_FT_V33 low speed @ 1.2V pullup"
io8_ft_v33_ls_pd_1v2  "IO8_FT_V33 low speed @ 1.2V pulldown"
io8_ft_v33_hs_1v8  "IO8_FT_V33 high speed @ 1.8V"
io8_ft_v33_hs_pu_1v8  "IO8_FT_V33 high speed @ 1.8V pullup"
io8_ft_v33_hs_pd_1v8  "IO8_FT_V33 high speed @ 1.8V pulldown"
io8_ft_v33_fs_1v8  "IO8_FT_V33 fast speed @ 1.8V"
io8_ft_v33_fs_pu_1v8  "IO8_FT_V33 fast speed @ 1.8V pullup"
io8_ft_v33_fs_pd_1v8  "IO8_FT_V33 fast speed @ 1.8V pulldown"
io8_ft_v33_ms_1v8  "IO8_FT_V33 med speed @ 1.8V"
io8_ft_v33_ms_pu_1v8  "IO8_FT_V33 med speed @ 1.8V pullup"
io8_ft_v33_ms_pd_1v8  "IO8_FT_V33 med speed @ 1.8V pulldown"
io8_ft_v33_ls_1v8  "IO8_FT_V33 low speed @ 1.8V"
io8_ft_v33_ls_pu_1v8  "IO8_FT_V33 low speed @ 1.8V pullup"
io8_ft_v33_ls_pd_1v8  "IO8_FT_V33 low speed @ 1.8V pulldown"
io8_ft_v33_hs_3v3  "IO8_FT_V33 high speed @ 3.3V"
io8_ft_v33_hs_pu_3v3  "IO8_FT_V33 high speed @ 3.3V pullup"
io8_ft_v33_hs_pd_3v3  "IO8_FT_V33 high speed @ 3.3V pulldown"
io8_ft_v33_fs_3v3  "IO8_FT_V33 fast speed @ 3.3V"
io8_ft_v33_fs_pu_3v3  "IO8_FT_V33 fast speed @ 3.3V pullup"
io8_ft_v33_fs_pd_3v3  "IO8_FT_V33 fast speed @ 3.3V pulldown"
io8_ft_v33_ms_3v3  "IO8_FT_V33 med speed @ 3.3V"
io8_ft_v33_ms_pu_3v3  "IO8_FT_V33 med speed @ 3.3V pullup"
io8_ft_v33_ms_pd_3v3  "IO8_FT_V33 med speed @ 3.3V pulldown"
io8_ft_v33_ls_3v3  "IO8_FT_V33 low speed @ 3.3V"
io8_ft_v33_ls_pu_3v3  "IO8_FT_V33 low speed @ 3.3V pullup"
io8_ft_v33_ls_pd_3v3  "IO8_FT_V33 low speed @ 3.3V pulldown"
[Model Selector] io8_usb_ft
io8_100m_ft_hs_1v2  "IO8_FT 100MHz high speed @ 1.2V"
io8_100m_ft_hs_pu_1v2  "IO8_FT 100MHz high speed @ 1.2V pullup"
io8_100m_ft_hs_pd_1v2  "IO8_FT 100MHz high speed @ 1.2V pulldown"
io8_100m_ft_fs_1v2  "IO8_FT 100MHz fast speed @ 1.2V"
io8_100m_ft_fs_pu_1v2  "IO8_FT 100MHz fast speed @ 1.2V pullup"
io8_100m_ft_fs_pd_1v2  "IO8_FT 100MHz fast speed @ 1.2V pulldown"
io8_100m_ft_ms_1v2  "IO8_FT 100MHz med speed @ 1.2V"
io8_100m_ft_ms_pu_1v2  "IO8_FT 100MHz med speed @ 1.2V pullup"
io8_100m_ft_ms_pd_1v2  "IO8_FT 100MHz med speed @ 1.2V pulldown"
io8_100m_ft_ls_1v2  "IO8_FT 100MHz low speed @ 1.2V"
io8_100m_ft_ls_pu_1v2  "IO8_FT 100MHz low speed @ 1.2V pullup"
io8_100m_ft_ls_pd_1v2  "IO8_FT 100MHz low speed @ 1.2V pulldown"
io8_100m_ft_hs_1v8  "IO8_FT 100MHz high speed @ 1.8V"
io8_100m_ft_hs_pu_1v8  "IO8_FT 100MHz high speed @ 1.8V pullup"
io8_100m_ft_hs_pd_1v8  "IO8_FT 100MHz high speed @ 1.8V pulldown"
io8_100m_ft_fs_1v8  "IO8_FT 100MHz fast speed @ 1.8V"
io8_100m_ft_fs_pu_1v8  "IO8_FT 100MHz fast speed @ 1.8V pullup"
io8_100m_ft_fs_pd_1v8  "IO8_FT 100MHz fast speed @ 1.8V pulldown"
io8_100m_ft_ms_1v8  "IO8_FT 100MHz med speed @ 1.8V"
io8_100m_ft_ms_pu_1v8  "IO8_FT 100MHz med speed @ 1.8V pullup"
io8_100m_ft_ms_pd_1v8  "IO8_FT 100MHz med speed @ 1.8V pulldown"
io8_100m_ft_ls_1v8  "IO8_FT 100MHz low speed @ 1.8V"
io8_100m_ft_ls_pu_1v8  "IO8_FT 100MHz low speed @ 1.8V pullup"
io8_100m_ft_ls_pd_1v8  "IO8_FT 100MHz low speed @ 1.8V pulldown"
io8_100m_ft_hs_3v3  "IO8_FT 100MHz high speed @ 3.3V"
io8_100m_ft_hs_pu_3v3  "IO8_FT 100MHz high speed @ 3.3V pullup"
io8_100m_ft_hs_pd_3v3  "IO8_FT 100MHz high speed @ 3.3V pulldown"
io8_100m_ft_fs_3v3  "IO8_FT 100MHz fast speed @ 3.3V"
io8_100m_ft_fs_pu_3v3  "IO8_FT 100MHz fast speed @ 3.3V pullup"
io8_100m_ft_fs_pd_3v3  "IO8_FT 100MHz fast speed @ 3.3V pulldown"
io8_100m_ft_ms_3v3  "IO8_FT 100MHz med speed @ 3.3V"
io8_100m_ft_ms_pu_3v3  "IO8_FT 100MHz med speed @ 3.3V pullup"
io8_100m_ft_ms_pd_3v3  "IO8_FT 100MHz med speed @ 3.3V pulldown"
io8_100m_ft_ls_3v3  "IO8_FT 100MHz low speed @ 3.3V"
io8_100m_ft_ls_pu_3v3  "IO8_FT 100MHz low speed @ 3.3V pullup"
io8_100m_ft_ls_pd_3v3  "IO8_FT 100MHz low speed @ 3.3V pulldown"
io8_usb_fs_3v3  "IOUSB fast speed @ 3.3V"
io8_usb_fs_pu1_3v3  "IO8USB fast speed @ 3.3V pullup1"
io8_usb_fs_pd1_3v3  "IOUSB fast speed @ 3.3V pulldown1"
io8_usb_ls_3v3  "IOUSB low speed @ 3.3V"
io8_usb_ls_pu1_3v3  "IOUSB low speed @ 3.3V pullup1"
io8_usb_ls_pd1_3v3  "IOUSB low speed @ 3.3V pulldown1"
io8_usb_fs_pu2_3v3  "IOUSB fast speed @ 3.3V pullup2"
io8_usb_fs_pd2_3v3  "IOUSB fast speed @ 3.3V pulldown2"
io8_usb_ls_pu2_3v3  "IOUSB low speed @ 3.3V pullup2"
io8_usb_ls_pd2_3v3  "IOUSB low speed @ 3.3V pulldown2"
[Model Selector] io8_166m_hslv_ft
io8_166m_ft_hs_1v2  "IO8_FT 166MHz high speed @ 1.2V"
io8_166m_ft_hs_pu_1v2  "IO8_FT 166MHz high speed @ 1.2V pullup"
io8_166m_ft_hs_pd_1v2  "IO8_FT 166MHz high speed @ 1.2V pulldown"
io8_166m_ft_fs_1v2  "IO8_FT 166MHz fast speed @ 1.2V"
io8_166m_ft_fs_pu_1v2  "IO8_FT 166MHz fast speed @ 1.2V pullup"
io8_166m_ft_fs_pd_1v2  "IO8_FT 166MHz fast speed @ 1.2V pulldown"
io8_166m_ft_ms_1v2  "IO8_FT 166MHz med speed @ 1.2V"
io8_166m_ft_ms_pu_1v2  "IO8_FT 166MHz med speed @ 1.2V pullup"
io8_166m_ft_ms_pd_1v2  "IO8_FT 166MHz med speed @ 1.2V pulldown"
io8_166m_ft_ls_1v2  "IO8_FT 166MHz low speed @ 1.2V"
io8_166m_ft_ls_pu_1v2  "IO8_FT 166MHz low speed @ 1.2V pullup"
io8_166m_ft_ls_pd_1v2  "IO8_FT 166MHz low speed @ 1.2V pulldown"
io8_166m_ft_hs_1v8  "IO8_FT 166MHz high speed @ 1.8V"
io8_166m_ft_hs_pu_1v8  "IO8_FT 166MHz high speed @ 1.8V pullup"
io8_166m_ft_hs_pd_1v8  "IO8_FT 166MHz high speed @ 1.8V pulldown"
io8_166m_ft_fs_1v8  "IO8_FT 166MHz fast speed @ 1.8V"
io8_166m_ft_fs_pu_1v8  "IO8_FT 166MHz fast speed @ 1.8V pullup"
io8_166m_ft_fs_pd_1v8  "IO8_FT 166MHz fast speed @ 1.8V pulldown"
io8_166m_ft_ms_1v8  "IO8_FT 166MHz med speed @ 1.8V"
io8_166m_ft_ms_pu_1v8  "IO8_FT 166MHz med speed @ 1.8V pullup"
io8_166m_ft_ms_pd_1v8  "IO8_FT 166MHz med speed @ 1.8V pulldown"
io8_166m_ft_ls_1v8  "IO8_FT 166MHz low speed @ 1.8V"
io8_166m_ft_ls_pu_1v8  "IO8_FT 166MHz low speed @ 1.8V pullup"
io8_166m_ft_ls_pd_1v8  "IO8_FT 166MHz low speed @ 1.8V pulldown"
io8_166m_ft_hs_3v3  "IO8_FT 166MHz high speed @ 3.3V"
io8_166m_ft_hs_pu_3v3  "IO8_FT 166MHz high speed @ 3.3V pullup"
io8_166m_ft_hs_pd_3v3  "IO8_FT 166MHz high speed @ 3.3V pulldown"
io8_166m_ft_fs_3v3  "IO8_FT 166MHz fast speed @ 3.3V"
io8_166m_ft_fs_pu_3v3  "IO8_FT 166MHz fast speed @ 3.3V pullup"
io8_166m_ft_fs_pd_3v3  "IO8_FT 166MHz fast speed @ 3.3V pulldown"
io8_166m_ft_ms_3v3  "IO8_FT 166MHz med speed @ 3.3V"
io8_166m_ft_ms_pu_3v3  "IO8_FT 166MHz med speed @ 3.3V pullup"
io8_166m_ft_ms_pd_3v3  "IO8_FT 166MHz med speed @ 3.3V pulldown"
io8_166m_ft_ls_3v3  "IO8_FT 166MHz low speed @ 3.3V"
io8_166m_ft_ls_pu_3v3  "IO8_FT 166MHz low speed @ 3.3V pullup"
io8_166m_ft_ls_pd_3v3  "IO8_FT 166MHz low speed @ 3.3V pulldown"
io8_166m_hslv_ft_hs_1v2  "IO8_FT 166MHz HSLV high speed @ 1.2V"
io8_166m_hslv_ft_hs_pu_1v2  "IO8_FT 166MHz HSLV high speed @ 1.2V pullup"
io8_166m_hslv_ft_hs_pd_1v2  "IO8_FT 166MHz HSLV high speed @ 1.2V pulldown"
io8_166m_hslv_ft_fs_1v2  "IO8_FT 166MHz HSLV fast speed @ 1.2V"
io8_166m_hslv_ft_fs_pu_1v2  "IO8_FT 166MHz HSLV fast speed @ 1.2V pullup"
io8_166m_hslv_ft_fs_pd_1v2  "IO8_FT 166MHz HSLV fast speed @ 1.2V pulldown"
io8_166m_hslv_ft_ms_1v2  "IO8_FT 166MHz HSLV med speed @ 1.2V"
io8_166m_hslv_ft_ms_pu_1v2  "IO8_FT 166MHz HSLV med speed @ 1.2V pullup"
io8_166m_hslv_ft_ms_pd_1v2  "IO8_FT 166MHz HSLV med speed @ 1.2V pulldown"
io8_166m_hslv_ft_ls_1v2  "IO8_FT 166MHz HSLV low speed @ 1.2V"
io8_166m_hslv_ft_ls_pu_1v2  "IO8_FT 166MHz HSLV low speed @ 1.2V pullup"
io8_166m_hslv_ft_ls_pd_1v2  "IO8_FT 166MHz HSLV low speed @ 1.2V pulldown"
io8_166m_hslv_ft_hs_1v8  "IO8_FT 166MHz HSLV high speed @ 1.8V"
io8_166m_hslv_ft_hs_pu_1v8  "IO8_FT 166MHz HSLV high speed @ 1.8V pullup"
io8_166m_hslv_ft_hs_pd_1v8  "IO8_FT 166MHz HSLV high speed @ 1.8V pulldown"
io8_166m_hslv_ft_fs_1v8  "IO8_FT 166MHz HSLV fast speed @ 1.8V"
io8_166m_hslv_ft_fs_pu_1v8  "IO8_FT 166MHz HSLV fast speed @ 1.8V pullup"
io8_166m_hslv_ft_fs_pd_1v8  "IO8_FT 166MHz HSLV fast speed @ 1.8V pulldown"
io8_166m_hslv_ft_ms_1v8  "IO8_FT 166MHz HSLV med speed @ 1.8V"
io8_166m_hslv_ft_ms_pu_1v8  "IO8_FT 166MHz HSLV med speed @ 1.8V pullup"
io8_166m_hslv_ft_ms_pd_1v8  "IO8_FT 166MHz HSLV med speed @ 1.8V pulldown"
io8_166m_hslv_ft_ls_1v8  "IO8_FT 166MHz HSLV low speed @ 1.8V"
io8_166m_hslv_ft_ls_pu_1v8  "IO8_FT 166MHz HSLV low speed @ 1.8V pullup"
io8_166m_hslv_ft_ls_pd_1v8  "IO8_FT 166MHz HSLV low speed @ 1.8V pulldown"
io8_166m_hslv_ft_hs_2v5  "IO8_FT 166MHz HSLV high speed @ 2.5V"
io8_166m_hslv_ft_hs_pu_2v5  "IO8_FT 166MHz HSLV high speed @ 2.5V pullup"
io8_166m_hslv_ft_hs_pd_2v5  "IO8_FT 166MHz HSLV high speed @ 2.5V pulldown"
io8_166m_hslv_ft_fs_2v5  "IO8_FT 166MHz HSLV fast speed @ 2.5V"
io8_166m_hslv_ft_fs_pu_2v5  "IO8_FT 166MHz HSLV fast speed @ 2.5V pullup"
io8_166m_hslv_ft_fs_pd_2v5  "IO8_FT 166MHz HSLV fast speed @ 2.5V pulldown"
io8_166m_hslv_ft_ms_2v5  "IO8_FT 166MHz HSLV med speed @ 2.5V"
io8_166m_hslv_ft_ms_pu_2v5  "IO8_FT 166MHz HSLV med speed @ 2.5V pullup"
io8_166m_hslv_ft_ms_pd_2v5  "IO8_FT 166MHz HSLV med speed @ 2.5V pulldown"
io8_166m_hslv_ft_ls_2v5  "IO8_FT 166MHz HSLV low speed @ 2.5V"
io8_166m_hslv_ft_ls_pu_2v5  "IO8_FT 166MHz HSLV low speed @ 2.5V pullup"
io8_166m_hslv_ft_ls_pd_2v5  "IO8_FT 166MHz HSLV low speed @ 2.5V pulldown"
[Model Selector] io8_166m_hslv_i2c_ft
io8_166m_ft_hs_1v2  "IO8_FT 166MHz high speed @ 1.2V"
io8_166m_ft_hs_pu_1v2  "IO8_FT 166MHz high speed @ 1.2V pullup"
io8_166m_ft_hs_pd_1v2  "IO8_FT 166MHz high speed @ 1.2V pulldown"
io8_166m_ft_fs_1v2  "IO8_FT 166MHz fast speed @ 1.2V"
io8_166m_ft_fs_pu_1v2  "IO8_FT 166MHz fast speed @ 1.2V pullup"
io8_166m_ft_fs_pd_1v2  "IO8_FT 166MHz fast speed @ 1.2V pulldown"
io8_166m_ft_ms_1v2  "IO8_FT 166MHz med speed @ 1.2V"
io8_166m_ft_ms_pu_1v2  "IO8_FT 166MHz med speed @ 1.2V pullup"
io8_166m_ft_ms_pd_1v2  "IO8_FT 166MHz med speed @ 1.2V pulldown"
io8_166m_ft_ls_1v2  "IO8_FT 166MHz low speed @ 1.2V"
io8_166m_ft_ls_pu_1v2  "IO8_FT 166MHz low speed @ 1.2V pullup"
io8_166m_ft_ls_pd_1v2  "IO8_FT 166MHz low speed @ 1.2V pulldown"
io8_166m_ft_hs_1v8  "IO8_FT 166MHz high speed @ 1.8V"
io8_166m_ft_hs_pu_1v8  "IO8_FT 166MHz high speed @ 1.8V pullup"
io8_166m_ft_hs_pd_1v8  "IO8_FT 166MHz high speed @ 1.8V pulldown"
io8_166m_ft_fs_1v8  "IO8_FT 166MHz fast speed @ 1.8V"
io8_166m_ft_fs_pu_1v8  "IO8_FT 166MHz fast speed @ 1.8V pullup"
io8_166m_ft_fs_pd_1v8  "IO8_FT 166MHz fast speed @ 1.8V pulldown"
io8_166m_ft_ms_1v8  "IO8_FT 166MHz med speed @ 1.8V"
io8_166m_ft_ms_pu_1v8  "IO8_FT 166MHz med speed @ 1.8V pullup"
io8_166m_ft_ms_pd_1v8  "IO8_FT 166MHz med speed @ 1.8V pulldown"
io8_166m_ft_ls_1v8  "IO8_FT 166MHz low speed @ 1.8V"
io8_166m_ft_ls_pu_1v8  "IO8_FT 166MHz low speed @ 1.8V pullup"
io8_166m_ft_ls_pd_1v8  "IO8_FT 166MHz low speed @ 1.8V pulldown"
io8_166m_ft_hs_3v3  "IO8_FT 166MHz high speed @ 3.3V"
io8_166m_ft_hs_pu_3v3  "IO8_FT 166MHz high speed @ 3.3V pullup"
io8_166m_ft_hs_pd_3v3  "IO8_FT 166MHz high speed @ 3.3V pulldown"
io8_166m_ft_fs_3v3  "IO8_FT 166MHz fast speed @ 3.3V"
io8_166m_ft_fs_pu_3v3  "IO8_FT 166MHz fast speed @ 3.3V pullup"
io8_166m_ft_fs_pd_3v3  "IO8_FT 166MHz fast speed @ 3.3V pulldown"
io8_166m_ft_ms_3v3  "IO8_FT 166MHz med speed @ 3.3V"
io8_166m_ft_ms_pu_3v3  "IO8_FT 166MHz med speed @ 3.3V pullup"
io8_166m_ft_ms_pd_3v3  "IO8_FT 166MHz med speed @ 3.3V pulldown"
io8_166m_ft_ls_3v3  "IO8_FT 166MHz low speed @ 3.3V"
io8_166m_ft_ls_pu_3v3  "IO8_FT 166MHz low speed @ 3.3V pullup"
io8_166m_ft_ls_pd_3v3  "IO8_FT 166MHz low speed @ 3.3V pulldown"
io8_166m_hslv_ft_hs_1v2  "IO8_FT 166MHz HSLV high speed @ 1.2V"
io8_166m_hslv_ft_hs_pu_1v2  "IO8_FT 166MHz HSLV high speed @ 1.2V pullup"
io8_166m_hslv_ft_hs_pd_1v2  "IO8_FT 166MHz HSLV high speed @ 1.2V pulldown"
io8_166m_hslv_ft_fs_1v2  "IO8_FT 166MHz HSLV fast speed @ 1.2V"
io8_166m_hslv_ft_fs_pu_1v2  "IO8_FT 166MHz HSLV fast speed @ 1.2V pullup"
io8_166m_hslv_ft_fs_pd_1v2  "IO8_FT 166MHz HSLV fast speed @ 1.2V pulldown"
io8_166m_hslv_ft_ms_1v2  "IO8_FT 166MHz HSLV med speed @ 1.2V"
io8_166m_hslv_ft_ms_pu_1v2  "IO8_FT 166MHz HSLV med speed @ 1.2V pullup"
io8_166m_hslv_ft_ms_pd_1v2  "IO8_FT 166MHz HSLV med speed @ 1.2V pulldown"
io8_166m_hslv_ft_ls_1v2  "IO8_FT 166MHz HSLV low speed @ 1.2V"
io8_166m_hslv_ft_ls_pu_1v2  "IO8_FT 166MHz HSLV low speed @ 1.2V pullup"
io8_166m_hslv_ft_ls_pd_1v2  "IO8_FT 166MHz HSLV low speed @ 1.2V pulldown"
io8_166m_hslv_ft_hs_1v8  "IO8_FT 166MHz HSLV high speed @ 1.8V"
io8_166m_hslv_ft_hs_pu_1v8  "IO8_FT 166MHz HSLV high speed @ 1.8V pullup"
io8_166m_hslv_ft_hs_pd_1v8  "IO8_FT 166MHz HSLV high speed @ 1.8V pulldown"
io8_166m_hslv_ft_fs_1v8  "IO8_FT 166MHz HSLV fast speed @ 1.8V"
io8_166m_hslv_ft_fs_pu_1v8  "IO8_FT 166MHz HSLV fast speed @ 1.8V pullup"
io8_166m_hslv_ft_fs_pd_1v8  "IO8_FT 166MHz HSLV fast speed @ 1.8V pulldown"
io8_166m_hslv_ft_ms_1v8  "IO8_FT 166MHz HSLV med speed @ 1.8V"
io8_166m_hslv_ft_ms_pu_1v8  "IO8_FT 166MHz HSLV med speed @ 1.8V pullup"
io8_166m_hslv_ft_ms_pd_1v8  "IO8_FT 166MHz HSLV med speed @ 1.8V pulldown"
io8_166m_hslv_ft_ls_1v8  "IO8_FT 166MHz HSLV low speed @ 1.8V"
io8_166m_hslv_ft_ls_pu_1v8  "IO8_FT 166MHz HSLV low speed @ 1.8V pullup"
io8_166m_hslv_ft_ls_pd_1v8  "IO8_FT 166MHz HSLV low speed @ 1.8V pulldown"
io8_166m_hslv_ft_hs_2v5  "IO8_FT 166MHz HSLV high speed @ 2.5V"
io8_166m_hslv_ft_hs_pu_2v5  "IO8_FT 166MHz HSLV high speed @ 2.5V pullup"
io8_166m_hslv_ft_hs_pd_2v5  "IO8_FT 166MHz HSLV high speed @ 2.5V pulldown"
io8_166m_hslv_ft_fs_2v5  "IO8_FT 166MHz HSLV fast speed @ 2.5V"
io8_166m_hslv_ft_fs_pu_2v5  "IO8_FT 166MHz HSLV fast speed @ 2.5V pullup"
io8_166m_hslv_ft_fs_pd_2v5  "IO8_FT 166MHz HSLV fast speed @ 2.5V pulldown"
io8_166m_hslv_ft_ms_2v5  "IO8_FT 166MHz HSLV med speed @ 2.5V"
io8_166m_hslv_ft_ms_pu_2v5  "IO8_FT 166MHz HSLV med speed @ 2.5V pullup"
io8_166m_hslv_ft_ms_pd_2v5  "IO8_FT 166MHz HSLV med speed @ 2.5V pulldown"
io8_166m_hslv_ft_ls_2v5  "IO8_FT 166MHz HSLV low speed @ 2.5V"
io8_166m_hslv_ft_ls_pu_2v5  "IO8_FT 166MHz HSLV low speed @ 2.5V pullup"
io8_166m_hslv_ft_ls_pd_2v5  "IO8_FT 166MHz HSLV low speed @ 2.5V pulldown"
io8_166m_i2c_ft_1v2  "IO8_FT 166MHz I2C @ 1.2V"
io8_166m_i2c_ft_pu_1v2  "IO8_FT 166MHz I2C @ 1.2V pullup"
io8_166m_i2c_ft_pd_1v2  "IO8_FT 166MHz I2C @ 1.2V pulldown"
io8_166m_i2c_ft_1v8  "IO8_FT 166MHz I2C @ 1.8V"
io8_166m_i2c_ft_pu_1v8  "IO8_FT 166MHz I2C @ 1.8V pullup"
io8_166m_i2c_ft_pd_1v8  "IO8_FT 166MHz I2C @ 1,8V pulldown"
io8_166m_i2c_ft_3v3  "IO8_FT 166MHz I2C @ 3.3V"
io8_166m_i2c_ft_pu_3v3  "IO8_FT 166MHz I2C HSLV @ 3.3V pullup"
io8_166m_i2c_ft_pd_3v3  "IO8_FT 166MHz I2C @ 3.3V pulldown"
[Model Selector] io8_100m_ft_v33
io8_ft_v33_hs_1v2  "IO8_FT_V33 high speed @ 1.2V"
io8_ft_v33_hs_pu_1v2  "IO8_FT_V33 high speed @ 1.2V pullup"
io8_ft_v33_hs_pd_1v2  "IO8_FT_V33 high speed @ 1.2V pulldown"
io8_ft_v33_fs_1v2  "IO8_FT_V33 fast speed @ 1.2V"
io8_ft_v33_fs_pu_1v2  "IO8_FT_V33 fast speed @ 1.2V pullup"
io8_ft_v33_fs_pd_1v2  "IO8_FT_V33 fast speed @ 1.2V pulldown"
io8_ft_v33_ms_1v2  "IO8_FT_V33 med speed @ 1.2V"
io8_ft_v33_ms_pu_1v2  "IO8_FT_V33 med speed @ 1.2V pullup"
io8_ft_v33_ms_pd_1v2  "IO8_FT_V33 med speed @ 1.2V pulldown"
io8_ft_v33_ls_1v2  "IO8_FT_V33 low speed @ 1.2V"
io8_ft_v33_ls_pu_1v2  "IO8_FT_V33 low speed @ 1.2V pullup"
io8_ft_v33_ls_pd_1v2  "IO8_FT_V33 low speed @ 1.2V pulldown"
io8_ft_v33_hs_1v8  "IO8_FT_V33 high speed @ 1.8V"
io8_ft_v33_hs_pu_1v8  "IO8_FT_V33 high speed @ 1.8V pullup"
io8_ft_v33_hs_pd_1v8  "IO8_FT_V33 high speed @ 1.8V pulldown"
io8_ft_v33_fs_1v8  "IO8_FT_V33 fast speed @ 1.8V"
io8_ft_v33_fs_pu_1v8  "IO8_FT_V33 fast speed @ 1.8V pullup"
io8_ft_v33_fs_pd_1v8  "IO8_FT_V33 fast speed @ 1.8V pulldown"
io8_ft_v33_ms_1v8  "IO8_FT_V33 med speed @ 1.8V"
io8_ft_v33_ms_pu_1v8  "IO8_FT_V33 med speed @ 1.8V pullup"
io8_ft_v33_ms_pd_1v8  "IO8_FT_V33 med speed @ 1.8V pulldown"
io8_ft_v33_ls_1v8  "IO8_FT_V33 low speed @ 1.8V"
io8_ft_v33_ls_pu_1v8  "IO8_FT_V33 low speed @ 1.8V pullup"
io8_ft_v33_ls_pd_1v8  "IO8_FT_V33 low speed @ 1.8V pulldown"
io8_ft_v33_hs_3v3  "IO8_FT_V33 high speed @ 3.3V"
io8_ft_v33_hs_pu_3v3  "IO8_FT_V33 high speed @ 3.3V pullup"
io8_ft_v33_hs_pd_3v3  "IO8_FT_V33 high speed @ 3.3V pulldown"
io8_ft_v33_fs_3v3  "IO8_FT_V33 fast speed @ 3.3V"
io8_ft_v33_fs_pu_3v3  "IO8_FT_V33 fast speed @ 3.3V pullup"
io8_ft_v33_fs_pd_3v3  "IO8_FT_V33 fast speed @ 3.3V pulldown"
io8_ft_v33_ms_3v3  "IO8_FT_V33 med speed @ 3.3V"
io8_ft_v33_ms_pu_3v3  "IO8_FT_V33 med speed @ 3.3V pullup"
io8_ft_v33_ms_pd_3v3  "IO8_FT_V33 med speed @ 3.3V pulldown"
io8_ft_v33_ls_3v3  "IO8_FT_V33 low speed @ 3.3V"
io8_ft_v33_ls_pu_3v3  "IO8_FT_V33 low speed @ 3.3V pullup"
io8_ft_v33_ls_pd_3v3  "IO8_FT_V33 low speed @ 3.3V pulldown"
[Define Package Model]  455-ufbga-5x5-64ldo-100mhz-230421
[Manufacturer]  unknown
[OEM]  unknown
[Description]  unknown
[Number Of Pins]  59
[Pin Numbers]
| Pin Name Terminal   Net Name   Starting Node   Ending Node
E1 | NRST
G2 | PA0
H2 | PA1
F3 | PA2
G3 | PA3
H3 | PA4
F4 | PA5
G4 | PA6
H4 | PA7
D7 | PA8
C7 | PA9
C6 | PA10
C8 | PA11
B8 | PA12
A8 | PA13
A7 | PA14
A6 | PA15
F5 | PB0
G5 | PB1
G6 | PB2
A5 | PB3
A4 | PB4
C4 | PB5
D3 | PB6
C3 | PB7
B3 | PB8
A3 | PB9
G7 | PB10
H8 | PB12
G8 | PB13
F8 | PB14
F7 | PB15
E3 | PC0
E2 | PC1
F2 | PC2
G1 | PC3
H5 | PC4
H6 | PC5
F6 | PC6
E7 | PC7
E8 | PC8
D8 | PC9
B7 | PC10
B6 | PC11
C5 | PC12
A2 | PC13
A1 | PC14-OSC32_IN
B1 | PC15-OSC32_OUT
B5 | PD2
C1 | PH0-OSC_IN
D1 | PH1-OSC_OUT
B4 | PH3-BOOT0
B2 | VBAT
H7 | VCAP
D2 | VDD
H1 | VDDA
E5 | VDDUSB
C2 | VSS
F1 | VSSA
|[Merged Pins]  D2
|E4  |  VDD
|E6  |  VDD
|[Merged Pins]  C2
|D4  |  VSS
|D5  |  VSS
|D6  |  VSS
[Model Data]
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[End Model Data]
[End Package Model]
| Models and submodels in the file (208): io8_100m_ft_hs_1v2 (I/O), io8_100m_ft_hs_pu_1v2 (I/O), io8_100m_ft_hs_pd_1v2 (I/O), io8_100m_ft_fs_1v2 (I/O), io8_100m_ft_fs_pu_1v2 (I/O), io8_100m_ft_fs_pd_1v2 (I/O), io8_100m_ft_ms_1v2 (I/O), io8_100m_ft_ms_pu_1v2 (I/O), io8_100m_ft_ms_pd_1v2 (I/O), io8_100m_ft_ls_1v2 (I/O), io8_100m_ft_ls_pu_1v2 (I/O), io8_100m_ft_ls_pd_1v2 (I/O), io8_100m_ft_hs_1v8 (I/O), io8_100m_ft_hs_pu_1v8 (I/O), io8_100m_ft_hs_pd_1v8 (I/O), io8_100m_ft_fs_1v8 (I/O), io8_100m_ft_fs_pu_1v8 (I/O), io8_100m_ft_fs_pd_1v8 (I/O), io8_100m_ft_ms_1v8 (I/O), io8_100m_ft_ms_pu_1v8 (I/O), io8_100m_ft_ms_pd_1v8 (I/O), io8_100m_ft_ls_1v8 (I/O), io8_100m_ft_ls_pu_1v8 (I/O), io8_100m_ft_ls_pd_1v8 (I/O), io8_100m_ft_hs_3v3 (I/O), io8_100m_ft_hs_pu_3v3 (I/O), io8_100m_ft_hs_pd_3v3 (I/O), io8_100m_ft_fs_3v3 (I/O), io8_100m_ft_fs_pu_3v3 (I/O), io8_100m_ft_fs_pd_3v3 (I/O), io8_100m_ft_ms_3v3 (I/O), io8_100m_ft_ms_pu_3v3 (I/O), io8_100m_ft_ms_pd_3v3 (I/O), io8_100m_ft_ls_3v3 (I/O), io8_100m_ft_ls_pu_3v3 (I/O), io8_100m_ft_ls_pd_3v3 (I/O), io8_100m_hslv_ft_hs_1v2 (I/O), io8_100m_hslv_ft_hs_pu_1v2 (I/O), io8_100m_hslv_ft_hs_pd_1v2 (I/O), io8_100m_hslv_ft_fs_1v2 (I/O), io8_100m_hslv_ft_fs_pu_1v2 (I/O), io8_100m_hslv_ft_fs_pd_1v2 (I/O), io8_100m_hslv_ft_ms_1v2 (I/O), io8_100m_hslv_ft_ms_pu_1v2 (I/O), io8_100m_hslv_ft_ms_pd_1v2 (I/O), io8_100m_hslv_ft_ls_1v2 (I/O), io8_100m_hslv_ft_ls_pu_1v2 (I/O), io8_100m_hslv_ft_ls_pd_1v2 (I/O), io8_100m_hslv_ft_hs_1v8 (I/O), io8_100m_hslv_ft_hs_pu_1v8 (I/O), io8_100m_hslv_ft_hs_pd_1v8 (I/O), io8_100m_hslv_ft_fs_1v8 (I/O), io8_100m_hslv_ft_fs_pu_1v8 (I/O), io8_100m_hslv_ft_fs_pd_1v8 (I/O), io8_100m_hslv_ft_ms_1v8 (I/O), io8_100m_hslv_ft_ms_pu_1v8 (I/O), io8_100m_hslv_ft_ms_pd_1v8 (I/O), io8_100m_hslv_ft_ls_1v8 (I/O), io8_100m_hslv_ft_ls_pu_1v8 (I/O), io8_100m_hslv_ft_ls_pd_1v8 (I/O), io8_100m_hslv_ft_hs_2v5 (I/O), io8_100m_hslv_ft_hs_pu_2v5 (I/O), io8_100m_hslv_ft_hs_pd_2v5 (I/O), io8_100m_hslv_ft_fs_2v5 (I/O), io8_100m_hslv_ft_fs_pu_2v5 (I/O), io8_100m_hslv_ft_fs_pd_2v5 (I/O), io8_100m_hslv_ft_ms_2v5 (I/O), io8_100m_hslv_ft_ms_pu_2v5 (I/O), io8_100m_hslv_ft_ms_pd_2v5 (I/O), io8_100m_hslv_ft_ls_2v5 (I/O), io8_100m_hslv_ft_ls_pu_2v5 (I/O), io8_100m_hslv_ft_ls_pd_2v5 (I/O), io8_166m_ft_hs_1v2 (I/O), io8_166m_ft_hs_pu_1v2 (I/O), io8_166m_ft_hs_pd_1v2 (I/O), io8_166m_ft_fs_1v2 (I/O), io8_166m_ft_fs_pu_1v2 (I/O), io8_166m_ft_fs_pd_1v2 (I/O), io8_166m_ft_ms_1v2 (I/O), io8_166m_ft_ms_pu_1v2 (I/O)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
